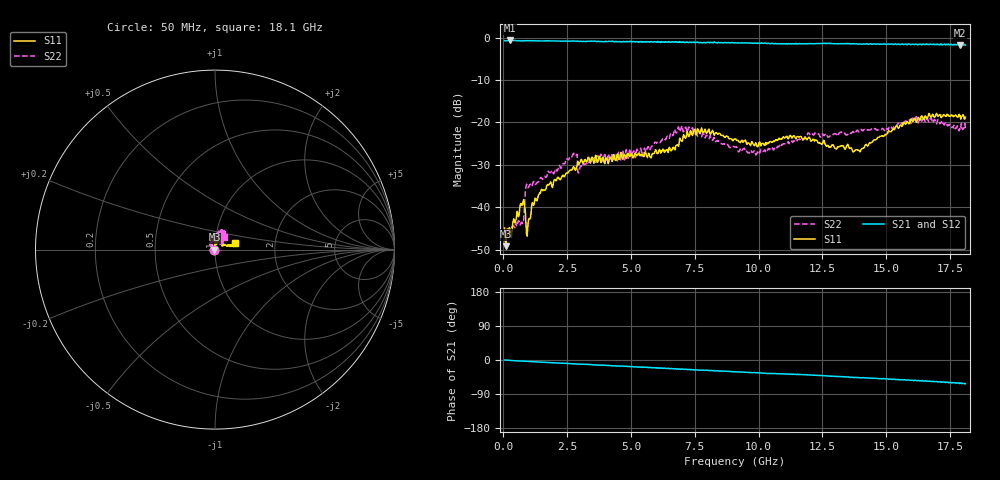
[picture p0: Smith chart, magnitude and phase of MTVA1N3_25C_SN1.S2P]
! Network Analyzer HP8720D.06.14 Serial No. US36140669
! 10 Jan 2005  13:42:50
! Frequency  S11  S21  S12  S22
# HZ  S  DB R 50
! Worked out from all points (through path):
!   801 points, 50 MHz to 18.1 GHz, reference 50 ohm
!   highest |S21| = -0.68 dB at 253.1 MHz (marker M1); lowest = -1.8 dB at 17.9 GHz (marker M2)
!   group delay of S21, straight-line fit = 9.17 ps
!   lowest |S11| = -49.2 dB at 95.12 MHz (marker M3), VSWR 1.01, Z = 49.7 - j0.00837 ohm
!   |S11| at or under -10 dB: start of sweep to end of sweep
!   |S22| runs from -48.0 to -18.6 dB; largest |S21 - S12| = 0.023
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5e7  -44.91 -141.6  -0.73 -0.1  -0.74 -0.4  -47.91 172.8
9.5125e7  -49.18 -178.6  -0.74 -0.5  -0.75 -0.8  -47.17 -170.5
2.530625e8  -44.98 152.9  -0.68 -0.9  -0.69 -1.2  -45.31 174.5
7.494375e8  -39.48 102.2  -0.76 -3.1  -0.76 -3.2  -43.84 163.6
9.750625e8  -43.45 108.2  -0.74 -3.8  -0.71 -4.0  -35.42 153.5
1.178125e9  -39.56 111.7  -0.73 -4.8  -0.74 -5.1  -33.99 140.5
1.471438e9  -36.15 106.5  -0.80 -5.6  -0.78 -5.8  -32.97 131.9
2.802625e9  -31.18 77.4  -0.84 -10.3  -0.82 -10.9  -27.84 122.3
3.005688e9  -29.44 87.9  -0.87 -11.1  -0.88 -11.2  -30.61 138.9
3.073375e9  -28.79 82.6  -0.87 -11.2  -0.83 -11.4  -30.41 136.3
5.510125e9  -28.07 80.3  -0.99 -19.5  -0.98 -19.6  -26.38 117.1
6.074188e9  -27.13 88.2  -1.01 -21.7  -1.01 -21.5  -24.55 108.7
7.066938e9  -22.86 94.0  -1.05 -25.0  -1.05 -24.7  -22.19 77.5
7.834062e9  -22.42 87.4  -1.16 -26.5  -1.11 -27.3  -22.68 53.5
9.075e9  -23.90 93.9  -1.25 -31.0  -1.19 -31.3  -25.79 46.1
9.954938e9  -25.72 99.6  -1.31 -33.5  -1.29 -34.2  -26.93 53.1
1.209838e10  -24.22 75.8  -1.41 -39.8  -1.40 -40.1  -22.71 74.3
1.392594e10  -26.63 29.5  -1.55 -46.4  -1.51 -46.6  -22.23 80.3
1.509919e10  -21.93 17.8  -1.54 -50.7  -1.45 -50.4  -21.39 81.0
1.640781e10  -18.54 14.4  -1.68 -54.3  -1.56 -54.8  -19.57 66.3
1.789694e10  -18.39 14.7  -1.81 -60.6  -1.86 -61.1  -21.77 61.7
1.81e10  -18.76 18.0  -1.78 -62.7  -1.73 -63.8  -21.50 54.0
